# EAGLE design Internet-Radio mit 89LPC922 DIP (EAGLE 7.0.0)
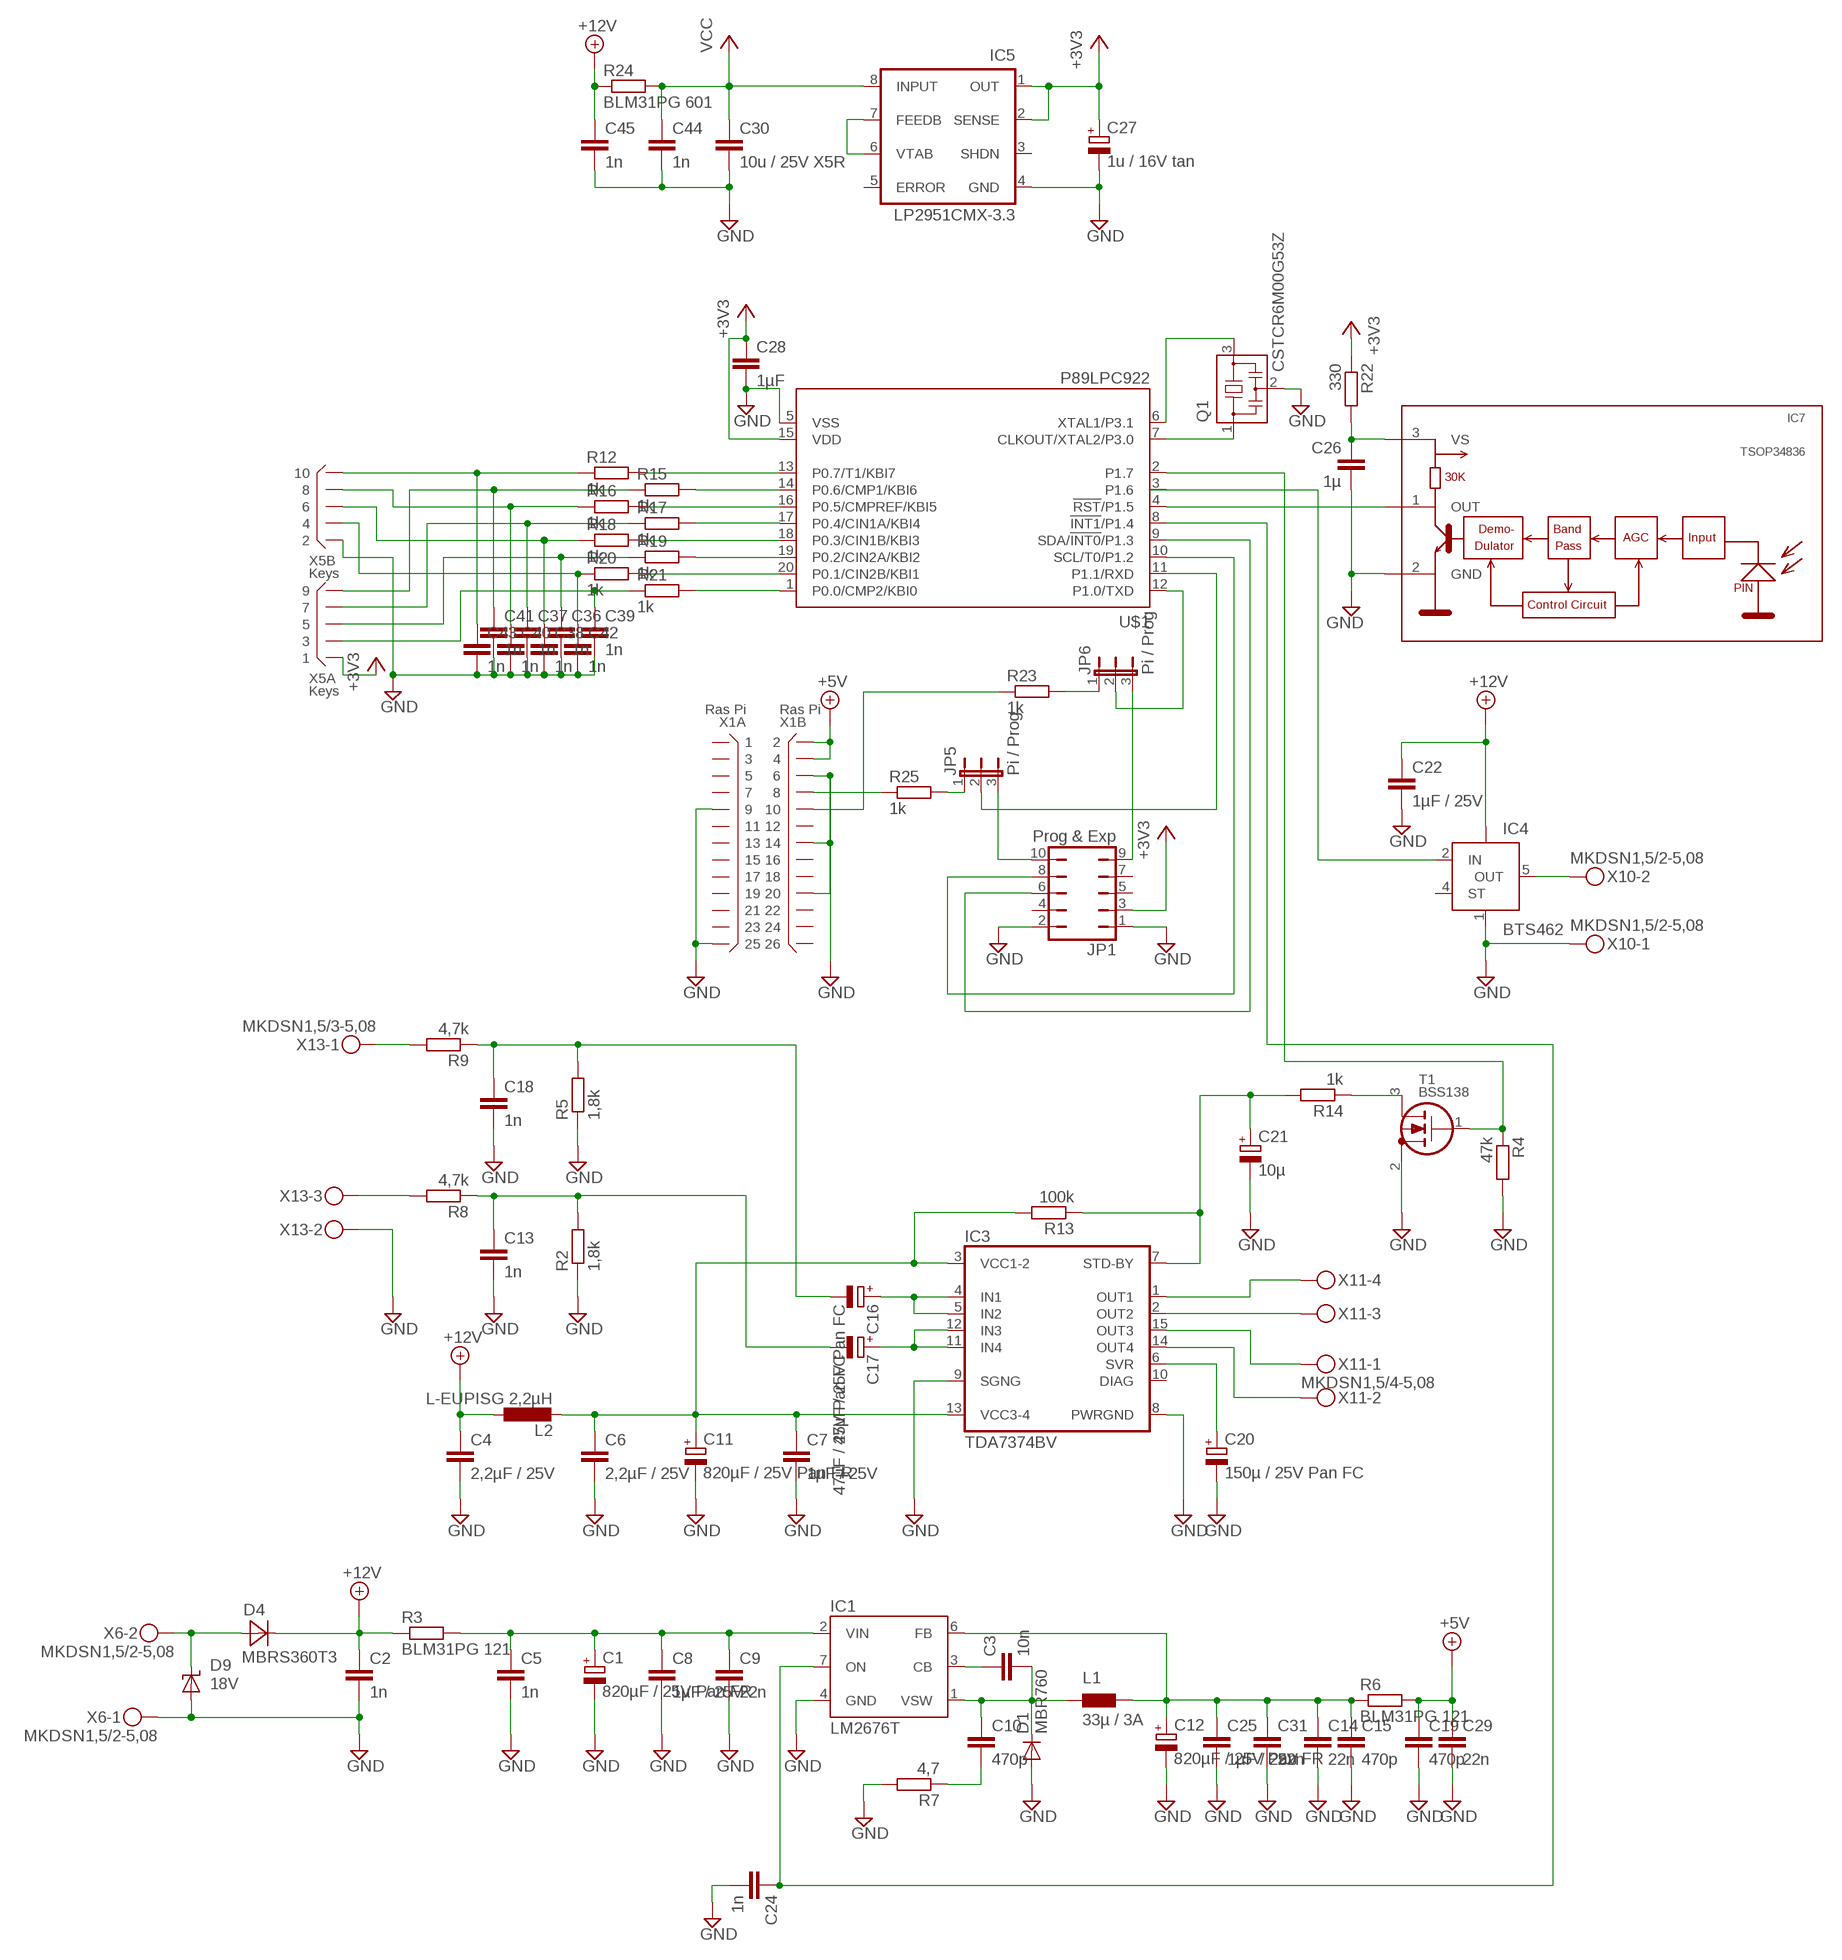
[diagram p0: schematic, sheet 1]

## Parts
C1  820µF / 25V Pan FR  CPOL-EUTT5D10  [TT5D10]
C2  1n  C-EUC0805  [C0805]
C3  10n  C-EUC0805  [C0805]
C4  2,2µF / 25V  C-EUC0805  [C0805]
C5  1n  C-EUC0805  [C0805]
C6  2,2µF / 25V  C-EUC0805  [C0805]
C7  1µF / 25V  C-EUC0805  [C0805]
C8  1µF / 25V  C-EUC0805  [C0805]
C9  22n  C-EUC0805  [C0805]
C10  470p  C-EUC0805  [C0805]
C11  820µF / 25V Pan FR  CPOL-EUTT5D10  [TT5D10]
C12  820µF / 25V Pan FR  CPOL-EUTT5D10  [TT5D10]
C13  1n  C-EUC0805  [C0805]
C14  22n  C-EUC0805  [C0805]
C15  470p  C-EUC0805  [C0805]
C16  47µF / 25V Pan FC  CPOL-EUE2.5-5  [E2,5-5]
C17  47µF / 25V Pan FC  CPOL-EUE2.5-5  [E2,5-5]
C18  1n  C-EUC0805  [C0805]
C19  470p  C-EUC0805  [C0805]
C20  150µ / 25V Pan FC  CPOL-EUE3.5-8  [E3,5-8]
C21  10µ  CPOL-EUE2.5-5  [E2,5-5]
C22  1µF / 25V  C-EUC0805  [C0805]
C24  1n  C-EUC0805  [C0805]
C25  1µF / 25V  C-EUC0805  [C0805]
C26  1µ  C-EUC0805  [C0805]
C27  1u / 16V tan  CPOL-EUCT3216  [CT3216]
C28  1µF  C-EUC0805  [C0805]
C29  22n  C-EUC0805  [C0805]
C30  10u / 25V X5R  C-EUC1206  [C1206]
C31  22n  C-EUC0805  [C0805]
C36  1n  C-EUC0603  [C0603]
C37  1n  C-EUC0603  [C0603]
C38  1n  C-EUC0603  [C0603]
C39  1n  C-EUC0603  [C0603]
C40  1n  C-EUC0603  [C0603]
C41  1n  C-EUC0603  [C0603]
C42  1n  C-EUC0603  [C0603]
C43  1n  C-EUC0603  [C0603]
C44  1n  C-EUC0805  [C0805]
C45  1n  C-EUC0805  [C0805]
D1  MBR760  DIODE-TO220V  [TO220ACS]
D4  MBRS360T3  [SMC]
D9  18V  SUPPRESSOR-SMBJ  [SMBJ]
IC1  LM2676T  [TO220-7]
IC3  TDA7374BV  [MULTIWATT-15V]
IC4  BTS462  BTS428L2  [TO252-5-11]
IC5  LP2951CMX-3.3  [SO-08]
IC7  TSOP34836  [TSOP348]
JP1  Prog & Exp  JP5Q  [JP5Q]
JP5  Pi / Prog  JP2E  [JP2]
JP6  Pi / Prog  JP2E  [JP2]
L1  33µ / 3A  PIS4728  [PIS4728]
L2  L-EUPISG 2,2µH  L-EUPISG  [PISG]
Q1  CSTCR6M00G53Z  [CSTCR6M]
R2  1,8k  R-EU_R1206  [R1206]
R3  BLM31PG 121  R-EU_R1206  [R1206]
R4  47k  R-EU_R1206  [R1206]
R5  1,8k  R-EU_R1206  [R1206]
R6  BLM31PG 121  R-EU_R1206  [R1206]
R7  4,7  R-EU_R1206  [R1206]
R8  4,7k  R-EU_R1206  [R1206]
R9  4,7k  R-EU_R1206  [R1206]
R12  1k  R-EU_R1206  [R1206]
R13  100k  R-EU_R1206  [R1206]
R14  1k  R-EU_R1206  [R1206]
R15  1k  R-EU_R1206  [R1206]
R16  1k  R-EU_R1206  [R1206]
R17  1k  R-EU_R1206  [R1206]
R18  1k  R-EU_R1206  [R1206]
R19  1k  R-EU_R1206  [R1206]
R20  1k  R-EU_R1206  [R1206]
R21  1k  R-EU_R1206  [R1206]
R22  330  R-EU_R1206  [R1206]
R23  1k  R-EU_R1206  [R1206]
R24  BLM31PG 601  R-EU_R1206  [R1206]
R25  1k  R-EU_R1206  [R1206]
T1  BSS138  [SOT23]
U$1  P89LPC922  [DIL20]
X1  Ras Pi  X13X2  [X26N-IDC]
X5  Keys  X05X2  [X10N-IDC]
X6  MKDSN1,5/2-5,08  [MKDSN1,5/2-5,08]
X10  MKDSN1,5/2-5,08  [MKDSN1,5/2-5,08]
X11  MKDSN1,5/4-5,08  [MKDSN1,5/4-5,08]
X13  MKDSN1,5/3-5,08  [MKDSN1,5/3-5,08]

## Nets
+3V3: C27.+ C28.1 IC5.1(OUT) IC5.2(SENSE) JP1.3 R22.1 U$1.15(VDD) X5.1
+5V: C19.1 C29.1 R6.2 X1.2 X1.4
+12V: C2.1 C4.1 C22.1 C45.1 D4.C IC4.TAB(VBB) L2.1 R3.1 R24.1
GND: C1.- C2.2 C4.2 C5.2 C6.2 C7.2 C8.2 C9.2 C11.- C12.- C13.2 C14.2 C15.2 C18.2 C19.2 C20.- C21.- C22.2 C24.2 C25.2 C26.2 C27.- C28.2 C29.2 C30.2 C31.2 C36.2 C37.2 C38.2 C39.2 C40.2 C41.2 C42.2 C43.2 C44.2 C45.2 D1.A D9.A IC1.4(GND) IC3.8(PWRGND) IC3.9(SGNG) IC4.1(GND) IC5.4(GND) IC7.2(GND) JP1.1 JP1.2 Q1.2 R2.1 R4.2 R5.1 R7.2 T1.2(S) U$1.5(VSS) X1.6 X1.9 X1.14 X1.20 X1.25 X5.2 X6.1 X10.1 X13.2
N$1: C1.+ C5.1 C8.1 C9.1 IC1.2(VIN) R3.2
N$2: C3.2 C10.1 D1.C IC1.1(VSW) L1.P$1
N$3: IC3.1(OUT1) X11.4
N$4: C3.1 IC1.3(CB)
N$5: IC3.2(OUT2) X11.3
N$6: IC3.15(OUT3) X11.1
N$7: IC3.14(OUT4) X11.2
N$8: C6.1 C7.1 C11.+ IC3.3(VCC1-2) IC3.13(VCC3-4) L2.2 R13.2
N$9: D4.A D9.C X6.2
N$10: C20.+ IC3.6(SVR)
N$11: JP1.10 JP5.3
N$12: C16.- C18.1 R5.2 R9.1
N$13: R9.2 X13.1
N$14: C13.1 C17.- R2.2 R8.1
N$15: C10.2 R7.1
N$16: R8.2 X13.3
N$17: C12.+ C14.1 C15.1 C25.1 C31.1 IC1.6(FB) L1.P$2 R6.1
N$18: C21.+ IC3.7(STD-BY) R13.1 R14.2
N$19: Q1.3 U$1.6(XTAL1/P3.1)
N$20: IC4.5(OUT) X10.2
N$21: Q1.1 U$1.7(CLKOUT/XTAL2/P3.0)
N$22: R21.2 U$1.1(P0.0/CMP2/KBI0)
N$23: R14.1 T1.3(D)
N$24: C16.+ IC3.4(IN1) IC3.5(IN2)
N$25: R4.1 T1.1(G) U$1.2(P1.7)
N$26: C17.+ IC3.11(IN4) IC3.12(IN3)
N$27: R19.2 U$1.19(P0.2/CIN2A/KBI2)
N$28: C24.1 IC1.7(ON) U$1.8(!INT1!/P1.4)
N$29: JP5.2 U$1.11(P1.1/RXD)
N$30: R17.2 U$1.17(P0.4/CIN1A/KBI4)
N$31: R15.2 U$1.14(P0.6/CMP1/KBI6)
N$32: R12.2 U$1.13(P0.7/T1/KBI7)
N$33: IC7.1(OUT) U$1.4(!RST!/P1.5)
N$34: R16.2 U$1.16(P0.5/CMPREF/KBI5)
N$35: R18.2 U$1.18(P0.3/CIN1B/KBI3)
N$36: R20.2 U$1.20(P0.1/CIN2B/KBI1)
N$37: JP6.2 U$1.12(P1.0/TXD)
N$38: JP1.8 U$1.10(SCL/T0/P1.2)
N$39: JP1.6 U$1.9(SDA/!INT0!/P1.3)
N$40: C26.1 IC7.3(VS) R22.2
N$41: IC5.6(VTAB) IC5.7(FEEDB)
N$42: C38.1 R18.1 X5.6
N$43: C36.1 R19.1 X5.5
N$44: C42.1 R20.1 X5.4
N$45: C39.1 R21.1 X5.3
N$46: C43.1 R12.1 X5.10
N$47: C41.1 R15.1 X5.9
N$48: C40.1 R16.1 X5.8
N$49: C37.1 R17.1 X5.7
N$51: JP5.1 R25.2
N$53: JP6.1 R23.2
N$54: R23.1 X1.10
N$55: R25.1 X1.8
N$58: IC4.2(IN) U$1.3(P1.6)
P1.0: JP1.9 JP6.3
VCC: C30.1 C44.1 IC5.8(INPUT) R24.2
Unconnected: IC3.10(DIAG) IC4.4(ST) IC5.3(SHDN) IC5.5(ERROR) JP1.4 JP1.5 JP1.7 X1.1 X1.3 X1.5 X1.7 X1.11 X1.12 X1.13 X1.15 X1.16 X1.17 X1.18 X1.19 X1.21 X1.22 X1.23 X1.24 X1.26

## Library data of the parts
C1 C11 C12 C16 C17 C20 C21 C27 = rcl:CPOL-EU: POLARIZED CAPACITOR, European symbol
C2-C10 C13-C15 C18 C19 C22 C24-C26 C28-C31 C36-C45 = rcl:C-EU: CAPACITOR, European symbol
D1 = diode:DIODE-: DIODE
D4 = diode:MBRS360T3: Surface Mount Schottky Power Rectifier
D9 = diode:SUPPRESSOR-: Suppressor diode
IC1 = v-reg-3:LM2676: National Semiconductor 3.0A "Simple Switcher"(c) 260kHz, Vout 1.2-37V, Vin 40V, 150mOhm DMOS switch, 50µA standby current
IC3 = st-tda737X:TDA7374B
IC4 = infineon:BTS428L2: Smart High-Side Power Switch One Channel: 60mOhm Status Feedback Source: Source: www.infineon.com .. BTS428L2_20030912.pdf; OC_FARNELL: unknown; OC_NEWARK: unknown
IC5 = v-reg:LP2951?*: Series of Adjustable Micropower Voltage Regulators Source: http://cache.national.com/ds/LP/LP2950.pdf
IC7 = vishay-1:TSOP348*: IR Receiver Modules for Remote Control Systems http://www.vishay.com/ir-receiver-modules/
JP1 = jumper:JP5Q: JUMPER
JP5 JP6 = jumper:JP2E: JUMPER
L1 = inductor-fastron:PIS4728: Fastron SMD Power Inductors
L2 = Inductor-Fastron (2):L-EU
Q1 = murata-filter:CSTCR: Resonator Source: murata.co.jp; MPN: CSTCR6M00G53-R0; OC_FARNELL: 1170434; OC_NEWARK: 25M8759
R2 R4 R5 R7-R9 R13 R14 R22 R23 R25 = rcl:R-EU_: RESISTOR, European symbol
R3 R6 R12 R15-R21 R24 = resistor:R-EU_: RESISTOR, European symbol
T1 = transistors:BSS138: BSS138: N-channel enhancement MOSFET (ON Semiconductor) 50V Uds, 200mA Id, 225mW Ptot, 3.5&Omega; Rdson
U$1 = 89LPC922:P89LPC922
X1 = connectors:X13X2: Connector 2x13 pins
X5 = connectors:X05X2: Connector 2x5 pins
X6 X10 = con-phoenix-508:MKDSN1,5/2-5,08: MKDSN 1,5/ 2-5,08 Printklemme; MPN: MKDSN 1,5/2-5.08; OC_FARNELL: 1792903; OC_NEWARK: 30M2397
X11 = con-phoenix-508:MKDSN1,5/4-5,08: MKDSN 1,5/ 4-5,08 Printklemme Nennstrom: 13,5 A Nennspannung: 250 V Rastermaß: 5,08 mm Polzahl: 4 Anschlussart: Schraubanschluss Montage: Löten Anschlussrichtung Leiter/Platine: 0 ° Artikelnummer: 1729144 Source: http://eshop.phoenixcontact.com .. 1729144.pdf
X13 = con-phoenix-508:MKDSN1,5/3-5,08: MKDSN 1,5/ 3-5,08 Printklemme Nennstrom: 13,5 A Nennspannung: 250 V Rastermaß: 5,08 mm Polzahl: 3 Anschlussart: Schraubanschluss Montage: Löten Anschlussrichtung Leiter/Platine: 0 ° Artikelnummer: 1729131 Source: http://eshop.phoenixcontact.com .. 1729131.pdf; MPN: SMKDSN1,5/3-5,08; OC_FARNELL: 1792904; OC_NEWARK: 70R0299

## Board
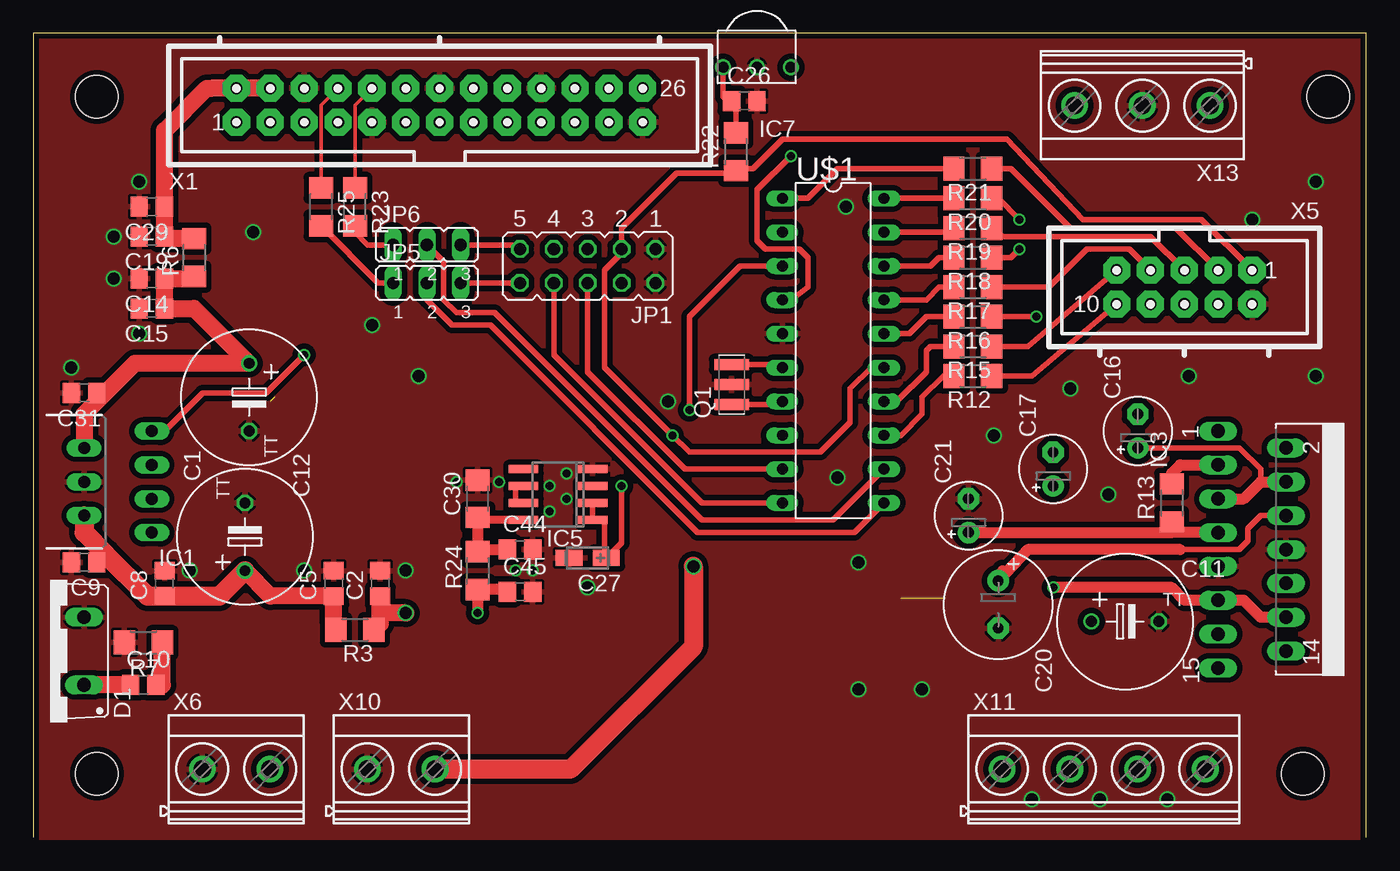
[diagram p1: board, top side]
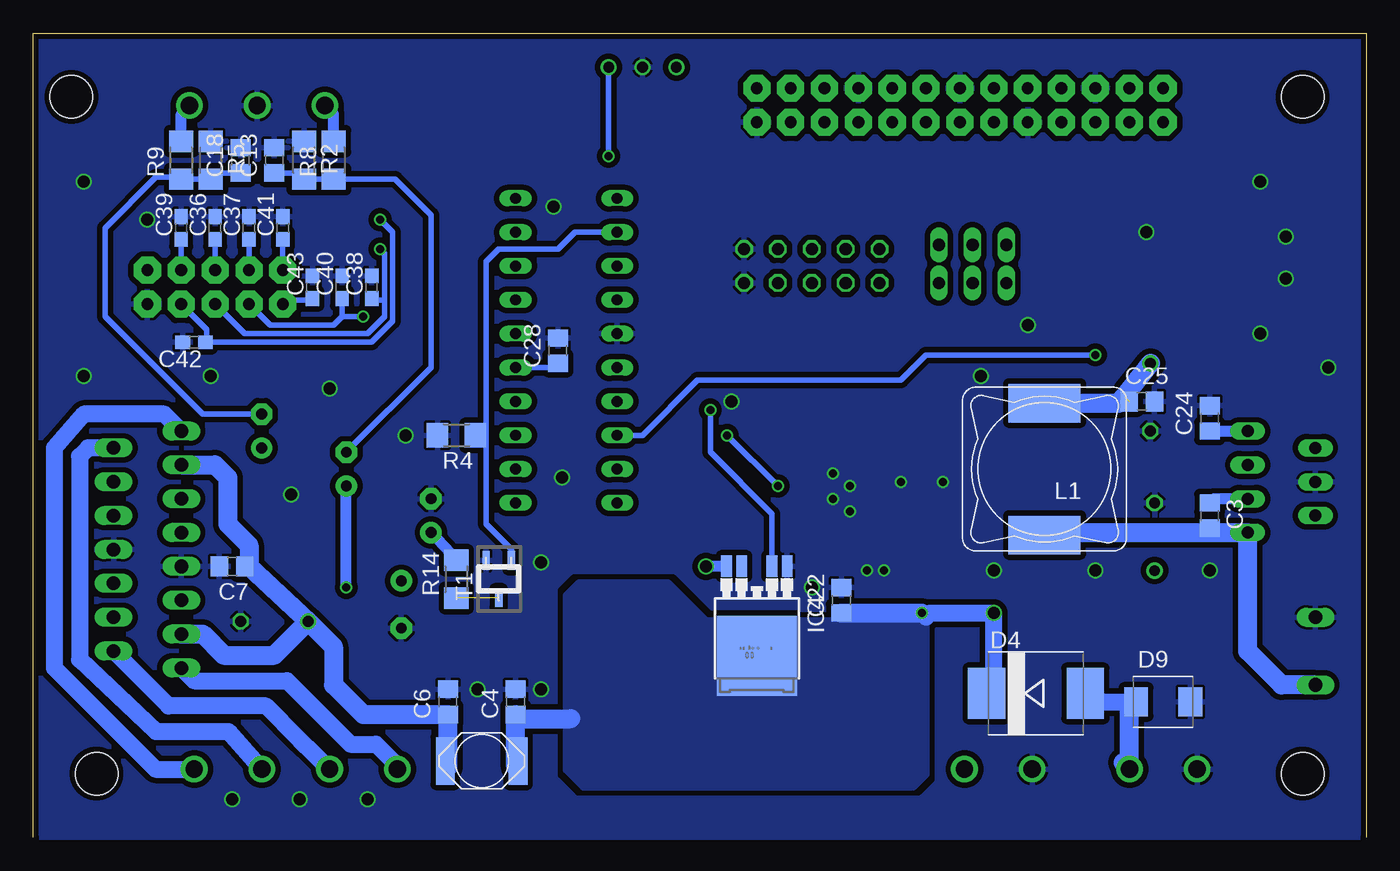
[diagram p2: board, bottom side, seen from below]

Size 100 x 60.33 mm. Coordinates in mm from the lower left corner, seen from the top.
Outline: 100,0 100,60.33 0,60.33 0,0
Copper layers (1*16): Top 0.035mm / dielectric 1.5mm / Bottom 0.035mm
Design rules "default": minimum track width 0.15mm, minimum drill 0.3mm, track to track 0.15mm, track to pad 0.15mm, pad to pad 0.15mm, via to via 0.15mm, smd to smd 0.15mm, copper to edge 0.3mm, drill to drill 0.2mm, minimum pad ring 0.2mm, minimum via ring 0.15mm, stop-mask expansion 0.075mm, vias tented up to drill 0mil, thermal gap 0.2mm
Holes 3.2 mm at 4.76,4.76 4.76,55.56 97.16,55.56 95.25,4.76

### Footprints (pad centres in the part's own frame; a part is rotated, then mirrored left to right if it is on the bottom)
TT5D10 = drill 0.813: + -2.54,0 | drill 0.813 octagon: - 2.54,0
C0805 = smd 1.3 x 1.5: 1 -0.95,0; 2 0.95,0
E2,5-5 = drill 0.813 pad 1.6: + -1.27,0 | drill 0.813 pad 1.6 octagon: - 1.27,0
E3,5-8 = drill 0.813 pad 1.6: + -1.778,0 | drill 0.813 pad 1.6 octagon: - 1.778,0
CT3216 = smd 2 x 1.2: + -1.4,0; - 1.4,0
C1206 = smd 1.6 x 1.8: 1 -1.4,0; 2 1.4,0
C0603 = smd 1.1 x 1: 1 -0.85,0; 2 0.85,0
TO220ACS = drill 1.016 long: A 2.54,-2.54; C -2.54,-2.54
SMC = smd 2.8 x 3.8: A 3.7,0; C -3.7,0
SMBJ = smd 1.78 x 2.16: A 2.04,0; C -2.03,0
TO220-7 = drill 0.9 long: 1 -3.81,-5.08; 2 -2.54,0; 3 -1.27,-5.08; 4 0,0; 5 1.27,-5.08; 6 2.54,0; 7 3.81,-5.08
MULTIWATT-15V = drill 1.016 long: 1 -8.89,-7.62; 2 -7.62,-2.54; 3 -6.35,-7.62; 4 -5.08,-2.54; 5 -3.81,-7.62; 6 -2.54,-2.54; 7 -1.27,-7.62; 8 0,-2.54; 9 1.27,-7.62; 10 2.54,-2.54; 11 3.81,-7.62; 12 5.08,-2.54; 13 6.35,-7.62; 14 7.62,-2.54; 15 8.89,-7.62
TO252-5-11 = smd 0.8 x 1.6: 1 -2.28,-5.41; 2 -1.14,-5.41; 4 1.14,-5.41; 5 2.28,-5.41 | smd 6 x 6: TAB 0,1.3
SO-08 = smd 0.6 x 2.2: 1 -1.905,-2.6; 2 -0.635,-2.6; 3 0.635,-2.6; 4 1.905,-2.6; 5 1.905,2.6; 6 0.635,2.6; 7 -0.635,2.6; 8 -1.905,2.6
TSOP348 = drill 0.8: 1 -2.54,0; 2 0,0; 3 2.54,0
JP5Q = drill 0.914 octagon: 1 -5.08,-1.27; 2 -5.08,1.27; 3 -2.54,-1.27; 4 -2.54,1.27; 5 0,-1.27; 6 0,1.27; 7 2.54,-1.27; 8 2.54,1.27; 9 5.08,-1.27; 10 5.08,1.27
JP2 = drill 0.914 long: 1 -2.54,0; 2 0,0; 3 2.54,0
PIS4728 = smd 5.4 x 2.9: P$1 0,4.95; P$2 0,-4.95
PISG = smd 1.4 x 3.56: 1 -2.73,0; 2 2.73,0
CSTCR6M = smd 0.8 x 2.6: 1 -1.5,0; 2 0,0; 3 1.5,0
R1206 = smd 1.6 x 1.803: 1 -1.422,0; 2 1.422,0
SOT23 = smd 0.55 x 1.4: 1 0.95,1.4; 2 -0.95,1.4; 3 0,-1.4
DIL20 = drill 0.813 long: 1 -11.43,-3.81; 2 -8.89,-3.81; 3 -6.35,-3.81; 4 -3.81,-3.81; 5 -1.27,-3.81; 6 1.27,-3.81; 7 3.81,-3.81; 8 6.35,-3.81; 9 8.89,-3.81; 10 11.43,-3.81; 11 11.43,3.81; 12 8.89,3.81; 13 6.35,3.81; 14 3.81,3.81; 15 1.27,3.81; 16 -1.27,3.81; 17 -3.81,3.81; 18 -6.35,3.81; 19 -8.89,3.81; 20 -11.43,3.81
X26N-IDC = drill 0.889 pad 2.032 octagon: 1 -15.24,-1.27; 2 -15.24,1.27; 3 -12.7,-1.27; 4 -12.7,1.27; 5 -10.16,-1.27; 6 -10.16,1.27; 7 -7.62,-1.27; 8 -7.62,1.27; 9 -5.08,-1.27; 10 -5.08,1.27; 11 -2.54,-1.27; 12 -2.54,1.27; 13 0,-1.27; 14 0,1.27; 15 2.54,-1.27; 16 2.54,1.27; 17 5.08,-1.27; 18 5.08,1.27; 19 7.62,-1.27; 20 7.62,1.27; 21 10.16,-1.27; 22 10.16,1.27; 23 12.7,-1.27; 24 12.7,1.27; 25 15.24,-1.27; 26 15.24,1.27
X10N-IDC = drill 0.889 pad 2.032 octagon: 1 -5.08,-1.27; 2 -5.08,1.27; 3 -2.54,-1.27; 4 -2.54,1.27; 5 0,-1.27; 6 0,1.27; 7 2.54,-1.27; 8 2.54,1.27; 9 5.08,-1.27; 10 5.08,1.27
MKDSN1,5/2-5,08 = drill 1.3 pad 2: 1 -2.561,0.025; 2 2.519,0.025
MKDSN1,5/4-5,08 = drill 1.3 pad 2: 1 -7.641,0.025; 2 -2.561,0.025; 3 2.519,0.025; 4 7.599,0.025
MKDSN1,5/3-5,08 = drill 1.3 pad 2: 1 -7.641,0.025; 2 -2.561,0.025; 3 2.519,0.025

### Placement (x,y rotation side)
C1  15.88,22.54 90 top
C2  26.04,19.05 90 top
C3  11.75,24.13 270 bottom
C4  63.82,10.16 90 bottom
C5  22.54,19.05 90 top
C6  68.9,10.16 90 bottom
C7  85.09,20.32 180 bottom
C8  9.84,19.05 90 top
C9  3.81,20.64 180 top
C10  8.26,11.43 0 top
C11  81.92,16.19 0 top
C12  16.19,33.02 270 top
C13  81.92,50.8 90 bottom
C14  8.89,41.91 180 top
C15  8.89,39.69 180 top
C16  82.87,30.48 90 top
C17  76.52,27.62 90 top
C18  84.45,50.8 90 bottom
C19  8.89,45.09 180 top
C20  72.39,17.46 270 top
C21  70.17,24.13 90 top
C22  39.37,17.78 90 bottom
C24  11.75,31.43 90 bottom
C25  16.83,32.7 0 bottom
C26  53.34,55.24 0 top
C27  41.59,20.95 180 top
C28  60.64,36.51 90 bottom
C29  8.89,47.31 180 top
C30  33.34,25.4 90 top
C31  3.81,33.34 180 top
C36  86.36,45.72 90 bottom
C37  83.82,45.72 90 bottom
C38  74.61,41.27 90 bottom
C39  88.9,45.72 90 bottom
C40  76.83,41.27 90 bottom
C41  81.28,45.72 90 bottom
C42  87.95,37.15 180 bottom
C43  79.06,41.27 90 bottom
C44  36.51,21.59 0 top
C45  36.51,18.41 0 top
D1  1.27,13.97 90 top
D4  24.77,10.79 0 bottom
D9  15.24,10.16 0 bottom
IC1  3.81,26.67 90 top
IC3  96.52,21.59 270 top
IC4  45.72,14.92 180 bottom
IC5  39.37,25.72 90 top
IC7  54.29,57.78 180 top
JP1  41.59,42.86 180 top
JP5  29.53,41.59 0 top
JP6  29.53,44.45 0 top
L1  24.13,27.62 180 bottom
L2  66.36,5.71 180 bottom
Q1  52.39,33.97 90 top
R2  79.69,50.8 270 bottom
R3  24.13,15.56 180 top
R4  68.26,30.16 180 bottom
R5  86.68,50.8 270 bottom
R6  12.06,43.5 90 top
R7  8.26,14.61 180 top
R8  77.47,50.8 90 bottom
R9  88.9,50.8 90 bottom
R12  70.48,34.61 180 top
R13  85.41,25.08 90 top
R14  68.26,19.37 90 bottom
R15  70.48,36.83 180 top
R16  70.48,39.05 180 top
R17  70.48,41.27 180 top
R18  70.48,43.5 180 top
R19  70.48,45.72 180 top
R20  70.48,47.94 180 top
R21  70.48,50.16 180 top
R22  52.7,51.44 90 top
R23  24.13,47.31 270 top
R24  33.34,20 90 top
R25  21.59,47.31 270 top
T1  65.09,19.37 0 bottom
U$1  60.01,36.51 270 top
X1  30.48,54.93 0 top
X5  86.36,41.27 180 top
X6  15.24,5.08 0 top
X10  27.62,5.08 0 top
X11  80.33,5.08 0 top
X13  80.64,54.93 180 top

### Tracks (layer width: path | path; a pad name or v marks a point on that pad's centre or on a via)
+3V3  (via drill 0.6)
  Top 0.406: IC5.2 IC5.1 42.86,23.81 42.86,21.59 C27.+ | C27.+ 43.18,20.95 | X5.1 87.63,46.35 78.74,46.35 73.03,52.39 56.2,52.39 53.98,50.16 52.86,50.16 R22.1 52.54,49.85 48.26,49.85 44.13,45.72 JP1.3 44.13,43.81 42.86,42.55 42.86,35.24 v47.94,30.16 49.21,28.89 59.05,28.89 61.28,31.11 61.28,33.66 62.87,35.24 U$1.15 | v44.13,26.35 44.13,22.09 C27.+
  Bottom 0.406: U$1.15 60.96,35.24 C28.1 | v47.94,30.16 v44.13,26.35
+5V
  Top 1.27: X1.4 X1.2 13.34,56.2 13.02,56.2 9.84,53.02 C29.1 C19.1 10.01,44.92 R6.2
+12V  (via drill 0.6, 0.9)
  Top 0.813: v33.34,16.83 R24.1 35.4,18.58 C45.1
  Top 1.27: R3.1 26.04,16.04 26.04,16.83 | 26.04,16.83 C2.1 | v27.94,16.83 26.04,16.83
  Bottom 0.813: v33.34,16.83 33.02,16.51 | L2.1 63.82,5.27 | C4.1 63.5,8.89
  Bottom 1.27: 33.02,16.51 32.7,16.83 v27.94,16.83 27.94,11.32 D4.C
  Bottom 1.422: C22.1 v33.34,16.83 | 63.82,5.27 C4.1 | 63.5,8.89 59.69,8.89
  pour Bottom (no thermals): 38.42,16.83 39.05,16.19 49.53,16.19 52.39,19.05 59.05,19.05 60.01,18.1 60.01,5.08 58.74,3.81 33.97,3.81 33.02,4.76 33.02,16.83
GND  (via drill 0.6, 0.9)
  other vias: 61.91,11.11 66.67,11.11 20.32,20 27.94,20 80.01,2.86 85.09,2.86 74.93,2.86 47.62,32.7 96.2,34.61 96.2,49.21 61.91,20.64 77.79,33.66 16.51,45.4 40.01,27.3 38.73,26.35 38.73,24.45 40.01,25.4 36.2,20 37.47,20 28.89,34.61 72.07,30.16 41.59,18.73 31.75,26.67 25.4,38.42 34.92,26.67 86.68,34.61 91.44,46.35 80.64,25.72 7.94,37.78 6.03,41.91 6.03,45.09 7.94,49.21 2.86,35.24 11.75,20 60.33,26.99 60.96,47.31
  pour Bottom (isolate 0.406, rank 2): 0,0 100.33,0 100.01,60.33 0,60.33
  pour Top (isolate 0.406): 0,60.33 100.01,60.33 100.33,0 0,0
N$1
  Top 1.27: R3.2 22.54,16.03 C5.1 17.78,18.1 C1.+ | C9.1 5.4,21.27
  Top 1.422: IC1.2 3.81,22.86 5.4,21.27 8.57,18.1 C8.1 11.43,18.1 13.97,18.1 C1.+
N$2
  Top 1.27: C10.1 D1.C
  Bottom 0.813: C3.2 11.43,22.86 IC1.1
  Bottom 1.422: D1.C 6.35,11.43 8.89,13.97 IC1.1 24,22.86 L1.P$1
N$3
  Bottom 1.27: IC3.1 90.17,31.75 96.2,31.75 98.42,29.21 98.42,12.7 90.83,5.11 X11.4
N$4
  Bottom 0.406: 11.43,25.4
  Bottom 0.813: IC1.3 11.43,25.4 | C3.1 11.43,25.4
N$5
  Bottom 1.27: X11.3 85.36,7.94 90.81,7.94 96.52,13.34 96.52,28.57 95.89,29.21 IC3.2
N$6
  Bottom 1.27: IC3.15 87.95,11.75 80.96,11.75 76.2,6.99 74.3,6.99 72.71,5.4 72.71,5.08 | X11.1 72.71,5.08 | 72.71,5.08
N$7
  Bottom 1.27: X11.2 77.79,5.13 80.01,7.3 82.55,9.84 89.85,9.84 IC3.14
N$8
  Top 0.813: R13.2 85.41,27.3 86.04,27.94 IC3.3
  Bottom 0.813: L2.2 68.9,5.27 | C7.1 83.82,20.32
  Bottom 1.422: 68.9,5.27 C6.1 75.25,9.21 77.47,11.43 77.47,14.29 C11.+ | IC3.3 86.36,27.94 85.41,26.99 85.41,23.5 83.82,21.91 83.82,20.32 C11.+ | IC3.13 87.31,15.24 85.72,13.65 81.92,13.65 C11.+
N$9
  Bottom 1.27: D4.A 20.43,10.16 D9.C
  Bottom 1.422: X6.2 17.78,5.13 | 17.78,5.13 17.78,9.84 17.46,10.16 D9.C 17.14,10.16 | 17.78,5.13 18.24,5.59
N$10
  Top 0.406: IC3.6 92.08,24.13 91.12,23.18 91.12,22.23 90.49,21.59 86.04,21.59
  Top 0.813: 86.04,21.59 74.61,21.59 C20.+ 72.71,20
N$11
  Top 0.406: JP1.10 JP5.3
N$12
  Bottom 0.406: C18.1 86.21,49.85 R5.2 R9.1 89.05,49.53 90.81,49.53 94.61,45.72 94.61,39.05 87.31,31.75 C16.-
N$13
  Bottom 0.813: R9.2 88.9,54.29 X13.1
N$14
  Bottom 0.406: C13.1 80.17,49.85 R2.2 R8.1 72.87,49.38 70.17,46.67 70.17,35.24 C17.-
N$15
  Top 1.27: C10.2 9.68,11.43 R7.1
N$16
  Bottom 0.813: R8.2 77.47,54.29 78.08,54.9 X13.3
N$17  (1 unrouted)
  Top 1.27: 4.76,32.7 7.62,35.56 C12.+ 12.06,39.69 C15.1 C14.1 11.9,41.91 R6.1 | IC1.6 3.81,31.75 4.76,32.7 | C31.1 4.76,32.7
  Bottom 0.813: 18.1,33.02 18.19,33.02
  Bottom 1.422: L1.P$2 18.55,32.57 18.19,33.02 C12.+
N$18
  Top 0.813: C21.+ 85.41,22.86 | 85.41,22.86 R13.1 | IC3.7 85.41,22.86
  Bottom 0.813: C21.+ R14.2
N$19
  Top 0.406: Q1.3 55.65,35.47 U$1.6
N$20  (via drill 0.9)
  Top 1.422: v49.53,20.32 49.53,14.29 40.3,5.1 X10.2
  Bottom 0.813: IC4.5 48.3,20.32 v49.53,20.32
N$21
  Top 0.406: Q1.1 55.65,32.47 U$1.7
N$22
  Top 0.406: R21.2 60.33,50.16 58.1,47.94 U$1.1
N$23  (1 unrouted)
N$24
  Top 0.406: C16.+ 90.49,29.21 92.08,27.62 92.08,26.67
  Top 0.813: IC3.5 90.81,25.4 92.08,26.67 IC3.4
N$25
  Bottom 0.406: T1.1 64.14,21.59 66.04,23.5 66.04,30.16 | 66.04,30.16 66.04,43.18 65.09,44.13 60.64,44.13 59.37,45.4 U$1.2 | R4.1 66.04,30.16
N$26  (via drill 0.6)
  Top 0.813: IC3.12 92.08,16.51 90.81,17.78 IC3.11 86.36,17.78 85.41,18.73 v76.52,18.73
  Bottom 0.813: v76.52,18.73 C17.+
N$27
  Top 0.406: U$1.19 68.75,45.4 R19.2
N$28  (via drill 0.6)
  Top 0.406: v20.32,36.2 17.46,33.34 12.7,33.34 9.84,30.48 IC1.7
  Bottom 0.406: v20.32,36.2 33.02,36.2 34.92,34.29 50.16,34.29 54.29,30.16 U$1.8
  Bottom 0.813: C24.1 11.43,30.48 IC1.7
N$29
  Top 0.406: JP5.2 29.53,40.32 31.43,38.42 34.29,38.42 49.85,22.86 61.59,22.86 U$1.11
N$30
  Top 0.406: R17.2 67.94,41.27 66.99,40.32 U$1.17
N$31
  Top 0.406: R15.2 67.31,36.83 66.99,36.51 66.99,34.92 64.77,32.7 U$1.14
N$32
  Top 0.406: R12.2 68.26,34.61 66.67,33.02 66.67,31.75 65.09,30.16 U$1.13
N$33  (via drill 0.6)
  Top 0.406: U$1.4 56.83,40.32 58.1,41.27 58.1,43.5 57.47,44.13 54.93,44.13 54.29,44.77 54.29,48.58 v56.83,51.12
  Bottom 0.406: v56.83,51.12 IC7.1
N$34
  Top 0.406: U$1.16 65.72,37.78 66.99,39.05 R16.2
N$35
  Top 0.406: R18.2 67.94,43.5 67.31,42.86 U$1.18
N$36
  Top 0.406: U$1.20 R20.2
N$37
  Top 0.406: JP6.2 30.8,43.18 30.8,40.32 31.75,39.37 34.61,39.37 50.16,23.81 60.01,23.81 U$1.12
N$38
  Top 0.406: JP1.8 39.05,36.2 50.16,25.08 U$1.10
N$39
  Top 0.406: U$1.9 48.9,27.62 41.59,34.92 JP1.6
N$40
  Top 0.406: R22.2 52.7,54.76 51.75,55.56 | IC7.3 51.75,55.56 | 51.75,55.56 C26.1
N$41
  Top 0.406: IC5.7 36.2,25.14 36.2,26.35 IC5.6
N$42  (via drill 0.6)
  Top 0.406: v73.98,44.13 73.34,43.5 R18.1
  Bottom 0.406: X5.6 84.14,37.78 74.93,37.78 73.66,39.05 73.66,40.32 | 73.66,40.32 73.66,43.81 v73.98,44.13 | C38.1 74.83,40.32 73.66,40.32
N$43
  Top 0.406: X5.5 83.82,45.09 72.71,45.09 72.07,45.72 R19.1
  Bottom 0.406: C36.1 X5.5
N$44  (via drill 0.6)
  Top 0.406: R20.1 72.39,47.94 v73.98,46.35
  Bottom 0.406: v73.98,46.35 73.03,45.4 73.03,38.73 74.61,37.15 87,37.15 | X5.4 87,38.1 87,37.15 | C42.1 87,37.15
N$45
  Top 0.406: X5.3 85.72,45.72 77.79,45.72 73.34,50.16 R21.1
  Bottom 0.406: C39.1 X5.3
N$46
  Top 0.406: X5.10 74.93,34.61 R12.1
  Bottom 0.406: X5.10 80.96,40.32 79.06,40.32 C43.1
N$47
  Top 0.406: X5.9 74.61,36.83 R15.1
  Bottom 0.406: X5.9 C41.1
N$48  (via drill 0.6)
  Top 0.406: v75.25,39.05 R16.1
  Bottom 0.406: X5.8 82.23,38.42 77.47,38.42 76.83,39.05 | 76.83,39.05 v75.25,39.05 | C40.1 76.83,39.05
N$49
  Top 0.406: R17.1 76.2,41.27 79.06,44.13 82.23,44.13 X5.7
  Bottom 0.406: C37.1 X5.7
N$51
  Top 0.406: JP5.1 25.88,41.59 R25.2
N$53
  Top 0.406: R23.2 24.13,45.4 25.08,44.45 JP6.1
N$54
  Top 0.254: X1.10 24.13,54.93 R23.1
N$55
  Top 0.254: X1.8 21.59,54.93 R25.1
N$58  (via drill 0.6)
  Top 0.406: v49.21,32.07 49.21,39.05 53.02,42.86 U$1.3
  Bottom 0.406: IC4.2 44.58,24.26 49.21,28.89 v49.21,32.07
P1.0
  Top 0.406: JP6.3 36.2,44.45 JP1.9
VCC
  Top 0.61: IC5.8 33.66,23.81 33.47,24 C30.1
  Top 0.813: C30.1 R24.2 33.5,21.59 C44.1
